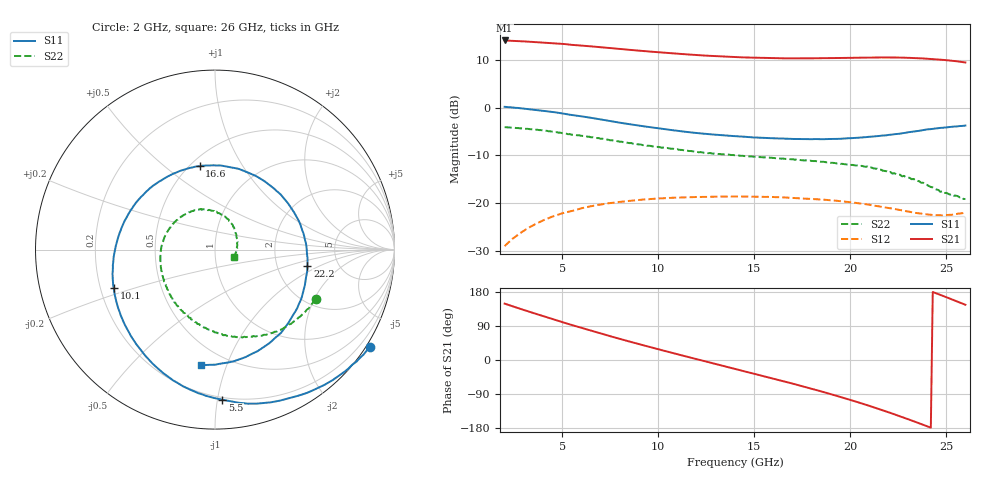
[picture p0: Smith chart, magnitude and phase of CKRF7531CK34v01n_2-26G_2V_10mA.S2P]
! CHUO DENSHI KOGYO Co.,Ltd.
! 14. January 2020
! CKRF7531CK34_RT5880
! N-channel HJ-FET
! Vds = 2 V, Id = 10 mA
# Hz S  MA  R 50
!	f	S11	S21	S12	S22
!	Hz	MAG	ANG	MAG	ANG	MAG	ANG	MAG	ANG
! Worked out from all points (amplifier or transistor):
!   241 points, 2 GHz to 26 GHz, reference 50 ohm
!   highest |S21| = 14.1 dB at 2 GHz (marker M1)
!   |S21| within 3 dB of that: start of sweep to 11.81 GHz
!   unconditionally stable (mu >= 1): 15.79 GHz to end of sweep
!   at 6 GHz: K = 0.47, MSG = 17.1 dB, |S12| = -21.1 dB
!   at 14 GHz: K = 0.94, MSG = 14.6 dB, |S12| = -18.6 dB
!   at 26 GHz: K = 1.26, MAG = 12.7 dB, |S12| = -22.0 dB
!   lowest NFmin = 0.59 dB at 18 GHz
!   S11 on the Smith chart (normalised r, x): 2 GHz: -0.13, -3.47; 5.5 GHz: 0.18, -1.03; 10.1 GHz: 0.26, -0.17; 16.6 GHz: 0.56, +0.67; 22.2 GHz: 2.99, -0.73; 26 GHz: 0.37, -0.82
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2e9  1.02 -32.1  5.06 148.8  0.03532 68.2  0.6251 -26.1
2.9e9  0.9825 -46.3  4.958 133.7  0.04976 57.4  0.6055 -36.8
3.8e9  0.9361 -60.5  4.841 119.0  0.06297 46.9  0.5815 -48.0
4.7e9  0.8894 -74.8  4.709 104.8  0.07458 36.7  0.5538 -59.1
5.5e9  0.8373 -87.2  4.552 92.3  0.08264 28.1  0.5205 -68.3
6e9  0.8099 -95.0  4.473 84.9  0.08805 23.2  0.5063 -74.0
8e9  0.6952 -126.5  4.123 55.7  0.103 3.4  0.439 -96.6
1e10  0.6075 -157.5  3.807 28.5  0.1115 -14.4  0.3877 -118.6
1.01e10  0.6035 -159.2  3.792 27.1  0.1121 -15.4  0.3841 -120.2
1.2e10  0.5417 171.7  3.56 2.2  0.1158 -31.6  0.3454 -140.9
1.4e10  0.5023 141.3  3.389 -23.3  0.1173 -48.3  0.3167 -162.4
1.66e10  0.4727 100.5  3.285 -57.0  0.1143 -71.9  0.2905 168.1
1.8e10  0.4671 76.6  3.289 -75.9  0.1103 -85.8  0.2762 151.3
1.91e10  0.4697 55.9  3.308 -91.7  0.1066 -98.6  0.2638 137.2
2.01e10  0.4791 35.9  3.325 -106.8  0.1016 -111.7  0.2512 122.5
2.11e10  0.4964 14.9  3.349 -122.7  0.09523 -126.8  0.2364 107.4
2.2e10  0.5176 -5.2  3.357 -138.0  0.08865 -142.5  0.2087 90.6
2.22e10  0.5224 -9.8  3.357 -141.5  0.08753 -146.6  0.2035 85.7
2.32e10  0.5571 -33.0  3.319 -159.7  0.08016 -168.6  0.1777 63.9
2.42e10  0.5954 -55.9  3.241 -178.6  0.07541 165.7  0.1474 39.1
2.51e10  0.6247 -76.1  3.13 163.9  0.07508 140.5  0.1253 9.1
2.6e10  0.6489 -96.8  2.975 145.8  0.07945 114.7  0.1104 -20.8
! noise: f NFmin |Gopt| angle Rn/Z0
1.8e+10  0.59  0.413  -118.9  0.07
1.85e+10  0.61  0.397  -111.2  0.08
1.9e+10  0.63  0.375  -103.2  0.09
2e+10  0.68  0.336  -85.9  0.12
2.05e+10  0.68  0.315  -76.4  0.13
2.1e+10  0.71  0.304  -66.6  0.14
2.2e+10  0.78  0.267  -46.2  0.15
2.25e+10  0.81  0.246  -35  0.16
2.3e+10  0.86  0.233  -18.1  0.17
2.4e+10  0.91  0.221  13  0.18
